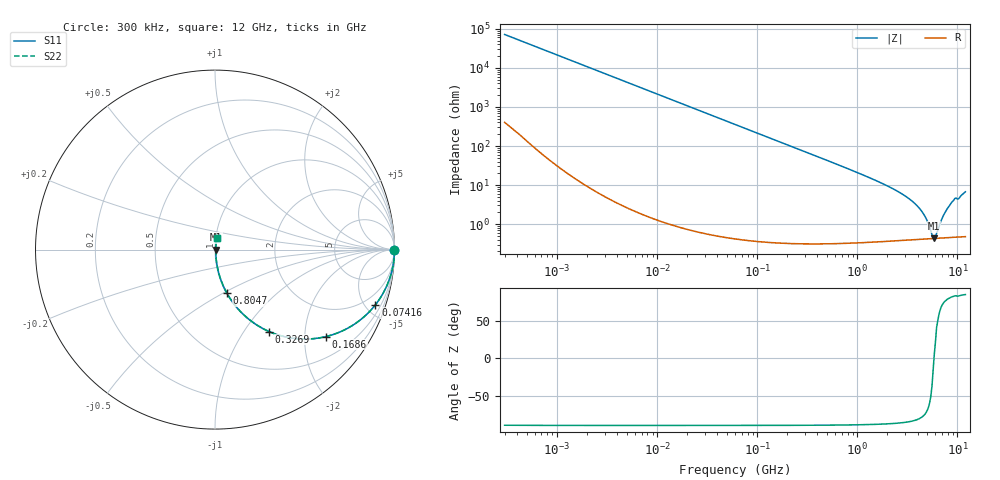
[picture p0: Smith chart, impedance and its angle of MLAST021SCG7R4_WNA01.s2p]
! MLAST021SCG7R4_WNA01  S-PARAMETER MODEL  ( General Type )
! Model Generated by TAIYO YUDEN Corporation (http://www.ty-top.com)
! Version 1.0
! TAIYO YUDEN Control No. 220901
! Copyright(c) 2022 TAIYO YUDEN CO.,LTD. All Rights Reserved.
! Product Description (link to TY-COMPAS)
! https://ds.yuden.co.jp/TYCOMPAS/or/detail?pn=MLAST021SCG7R4CWNA01&u=M
! Products Name : Multilayer Ceramic Capacitors
! Characteristics :
!  Capacitance : 7.4 pF , Rated Voltage : 25V , TCC : CG / C0G
!  Case Size : 0.25 x 0.125 / 0.0098 x 0.0049 [mm/inch] , Thickness : 0.125 / 0.0049 [mm/inch]
!  (Conditions: Temperature = 25 degC , DC Bias Current/Voltage = 0A / 0V)
! External Node Assignments :
!  1  o---| |---o  2
! GND o---------o GND
! Frequency Range : 0.3MHz  -  12000MHz  [ 401 STEP ]
# MHz S RI R 50
! Freq[MHz].  S11 Real  S11 Imag  S21 Real  S21 Imag  S12 Real  S12 Imag  S22 Real  S22 Imag
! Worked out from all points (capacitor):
!   401 points, 300 kHz to 12 GHz, reference 50 ohm
!   read as one part in series: C = 7.4 pF near 316.3 kHz
!   lowest |Z| = 432 mohm at 5.869 GHz (marker M1)
!   series resonance near 5.831 GHz, so ESL is about 100 pH
!   S11 on the Smith chart (normalised r, x): 300 kHz: open; 74.16 MHz: 1.01, -5.80; 168.6 MHz: 1.01, -2.55; 326.9 MHz: 1.01, -1.31; 804.7 MHz: 1.01, -0.52; 12 GHz: 1.01, +0.13
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0.3  1 -0.00139  9.81e-06 0.00139  9.81e-06 0.00139  1 -0.00139
1.769972  0.9999 -0.00823  7.53e-05 0.00823  7.53e-05 0.00823  0.9999 -0.00823
10.44266  0.9976 -0.0484  0.00238 0.0484  0.00238 0.0484  0.9976 -0.0484
27.10171  0.9843 -0.124  0.0157 0.124  0.0157 0.124  0.9843 -0.124
60  0.9275 -0.2587  0.0725 0.2587  0.0725 0.2587  0.9275 -0.2587
74.16388  0.8934 -0.308  0.1066 0.308  0.1066 0.308  0.8934 -0.308
110.3493  0.7911 -0.4056  0.2089 0.4056  0.2089 0.4056  0.7911 -0.4056
168.5979  0.6187 -0.4844  0.3813 0.4844  0.3813 0.4844  0.6187 -0.4844
326.9496  0.3016 -0.4566  0.6984 0.4566  0.6984 0.4566  0.3016 -0.4566
353.9943  0.2692 -0.441  0.7308 0.441  0.7308 0.441  0.2692 -0.441
804.7407  0.0669 -0.2438  0.9331 0.2438  0.9331 0.2438  0.0669 -0.2438
2088.533  0.0115 -0.0883  0.9885 0.0883  0.9885 0.0883  0.0115 -0.0883
3107.553  0.00628 -0.0489  0.9937 0.0489  0.9937 0.0489  0.00628 -0.0489
4050.141  0.00478 -0.0271  0.9952 0.0271  0.9952 0.0271  0.00478 -0.0271
4747.894  0.00437 -0.015  0.9956 0.015  0.9956 0.015  0.00437 -0.015
5565.855  0.00426 -0.0032  0.9957 0.0032  0.9957 0.0032  0.00426 -0.0032
5868.704  0.00428 0.000412  0.9957 -0.000412  0.9957 -0.000412  0.00428 0.000412
6188.031  0.00433 0.00385  0.9957 -0.00385  0.9957 -0.00385  0.00433 0.00385
7254.098  0.00468 0.0161  0.9953 -0.0161  0.9953 -0.0161  0.00468 0.0161
8281.503  0.00533 0.0286  0.9947 -0.0286  0.9947 -0.0286  0.00533 0.0286
9207.246  0.00626 0.0408  0.9937 -0.0408  0.9937 -0.0408  0.00626 0.0408
12000  0.00918 0.0662  0.9908 -0.0662  0.9908 -0.0662  0.00918 0.0662
